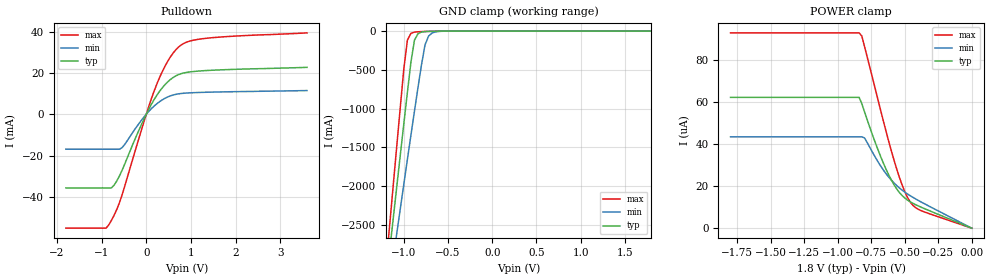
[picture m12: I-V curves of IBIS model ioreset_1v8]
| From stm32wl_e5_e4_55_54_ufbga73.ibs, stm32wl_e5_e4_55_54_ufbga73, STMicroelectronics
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|   Model ioreset_1v8
[Model]  ioreset_1v8
Model_type I/O_open_drain
Polarity   Inverting
Enable   Active-High
Vinl =   0.540000V
Vinh =   1.260000V
Vmeas =  0.900000V
Cref =   100.000000nF
Rref =   1.000000k
Vref =   1.800000V
C_comp   0.473010pF   0.460860pF   0.564710pF
[Temperature Range]   25.000000   0.125000k   -40.000000
[Pullup Reference]   1.800000V   1.600000V   2.000000V
[Pulldown Reference]   0.0V   0.0V   0.0V
[POWER Clamp Reference]   1.800000V   1.600000V   2.000000V
[GND Clamp Reference]   0.0V   0.0V   0.0V
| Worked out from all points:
|   slope of the pulldown table from 0 to 0.27 V, typ, clamps not added: 26.4 ohm
|   GND clamp passes 1 mA (typ) near -0.60 V on its own axis
[Pulldown]
|Voltage   I(typ)   I(min)   I(max)
-1.8V     -35.57mA   -16.85mA   -55.04mA
-900mV    -35.57mA   -16.85mA   -55.04mA
-840mV    -35.57mA   -16.85mA   -53.46mA
-720mV    -34.24mA   -16.85mA   -48.8mA
-540mV    -26.98mA   -16.06mA   -38.83mA
-60mV     -2.693mA   -1.52mA    -4.162mA
240mV     9.344mA    5.185mA    14.82mA
480mV     15.7mA     8.411mA    25.67mA
720mV     19.21mA    9.912mA    32.49mA
960mV     20.48mA    10.39mA    35.34mA
1.32V     21.16mA    10.68mA    36.74mA
3.6V      22.74mA    11.51mA    39.4mA
[GND_clamp]
|Voltage   I(typ)   I(min)   I(max)
-1.8V     -9.477A    -8.509A    -9.704A
-1.2V     -3.243A    -3.574A    -3.012A
-1.16V    -2.83A     -3.252A    -2.501A
-1.12V    -2.418A    -2.932A    -1.991A
-1.08V    -2.008A    -2.612A    -1.484A
-1V       -1.194A    -1.975A    -486.6mA
-960mV    -792.8mA   -1.659A    -118.4mA
-920mV    -402mA     -1.345A    -29.21mA
-880mV    -117.9mA   -1.034A    -12.85mA
-760mV    -5.956mA   -176.1mA   -5.379mA
-680mV    -2.455mA   -23.94mA   -2.76mA
1.8V      0A         0A         0A
[POWER_clamp]
|Voltage   I(typ)   I(min)   I(max)
-1.8V     62.29uA    43.51uA    93.01uA
-840mV    62.29uA    43.51uA    93.01uA
-820mV    59.25uA    43.51uA    91.5uA
-800mV    55.41uA    42.97uA    86.53uA
-700mV    37.44uA    31.68uA    61.29uA
-620mV    25.45uA    24.39uA    41.51uA
-580mV    20.7uA     21.55uA    32.43uA
-540mV    17.01uA    19.18uA    24.28uA
-480mV    13.41uA    16.32uA    14.73uA
-440mV    11.87uA    14.72uA    10.94uA
-400mV    10.63uA    13.26uA    9.03uA
0V        0A         0A         0A
[Ramp]
| variable   typ   min   max
dV/dt_r  1.07940/0.30020u   0.95906/0.30011u   1.19957/0.30008u
dV/dt_f  1.07940/13.44591n   0.95906/23.73127n   1.19957/9.52461n
R_load = 40.000000k
